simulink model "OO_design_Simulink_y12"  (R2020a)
settings: Solver=ode45  StartTime=0.0  StopTime=100  RelTol=1e-3  EnableMultiTasking=on
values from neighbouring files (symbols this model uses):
  Ao1 = Am-K1*Cm(1,:)    [OO_design.m]    (also in OO_design_y12.m = Am - K1*Cm(1,:))
  Ao2 = Am-K2*Cm(2,:)    [OO_design.m]    (also in OO_design_y12.m = Am - K2*Cm(2,:))
  Bo1 = [Bm K1]    [OO_design.m]    (also in OO_design_y12.m)
  Bo2 = [Bm-K2*Dm(2,1) K2]    [OO_design.m]    (also in OO_design_y12.m)
  Co1 = Cm(1,:)    [OO_design.m]    (also in OO_design_y12.m)
  Co2 = Cm(2,:)    [OO_design.m]    (also in OO_design_y12.m)
  Do1 = zeros(1,2)    [OO_design.m]    (also in OO_design_y12.m)
  Do2 = [Dm(2,1) 0]    [OO_design.m]    (also in OO_design_y12.m)
  Ts = 0.05    [init_model.m]

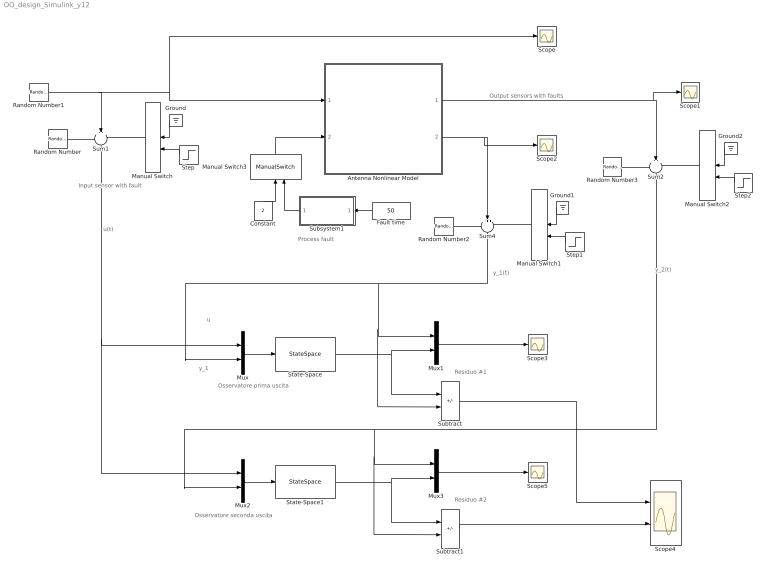
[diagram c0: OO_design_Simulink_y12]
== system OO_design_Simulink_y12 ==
  note: Osservatore seconda uscita
  note: Residuo #2
  note: Residuo #1
  note: Osservatore prima uscita
  note: y_1
  note: u
  note: u(t)
  note: Output sensors with faults
  note: Process fault
  note: Input sensor with fault
  note: y_1(t)
  note: y_2(t)
  Antenna Nonlinear Model : Subsystem
  Constant : Constant  Value=2
  Fault time : Constant  Value=50
  Ground : Ground
  Ground1 : Ground
  Ground2 : Ground
  Manual Switch{,1..3} (4 alike) : ManualSwitch
  Mux{,1..3} (4 alike) : Mux  Inputs=2
  Random Number : RandomNumber  Variance=0.0001  Seed=1  SampleTime=Ts
  Random Number1 : RandomNumber  Variance=0.1  SampleTime=10
  Random Number2 : RandomNumber  Variance=0.00001  Seed=2  SampleTime=Ts
  Random Number3 : RandomNumber  Variance=0.00001  Seed=3  SampleTime=Ts
  Scope{,1..3,5} (5 alike) : Scope
  Scope4 : Scope  NumInputPorts=2
  State-Space : StateSpace  A=Ao1  B=Bo1  C=Co1  D=Do1  InitialCondition=0
  State-Space1 : StateSpace  A=Ao2  B=Bo2  C=Co2  D=Do2  InitialCondition=0
  Step : Step  Time=50  SampleTime=0
  Step1 : Step  Time=50  SampleTime=0
  Step2 : Step  Time=50  SampleTime=0
  Subsystem1 : Subsystem
  Subtract : Sum  Inputs=+-
  Subtract1 : Sum  Inputs=+-
  Sum1 : Sum  Inputs=+++  SaturateOnIntegerOverflow=on
  Sum2 : Sum  Inputs=+++  SaturateOnIntegerOverflow=on
  Sum4 : Sum  Inputs=+++  SaturateOnIntegerOverflow=on
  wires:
  Random Number1/1 -> Scope/1, Antenna Nonlinear Model/1(force), Sum1/2
  Random Number/1 -> Sum1/1
  Manual Switch/1 -> Sum1/3
  Sum1/1 -> Mux2/1, Mux/1
  Ground/1 -> Manual Switch/1
  Step/1 -> Manual Switch/2
  Random Number2/1 -> Sum4/1
  Sum4/1 -> Mux1/1, Subtract/2, Mux/2
  Ground1/1 -> Manual Switch1/1
  Manual Switch1/1 -> Sum4/3
  Step1/1 -> Manual Switch1/2
  Antenna Nonlinear Model/2(velocity) -> Sum4/2, Scope2/1
  Random Number3/1 -> Sum2/1
  Ground2/1 -> Manual Switch2/1
  Manual Switch2/1 -> Sum2/3
  Step2/1 -> Manual Switch2/2
  Antenna Nonlinear Model/1(angle) -> Sum2/2, Scope1/1
  Sum2/1 -> Mux3/1, Subtract1/2, Mux2/2
  Fault time/1 -> Subsystem1/1(Fault time)
  Subsystem1/1(Fault) -> Manual Switch3/2
  Manual Switch3/1 -> Antenna Nonlinear Model/2(drag)
  Constant/1 -> Manual Switch3/1
  Mux/1 -> State-Space/1
  State-Space/1 -> Subtract/1, Mux1/2
  Subtract/1 -> Scope4/1
  Mux1/1 -> Scope3/1
  Mux2/1 -> State-Space1/1
  State-Space1/1 -> Subtract1/1, Mux3/2
  Mux3/1 -> Scope5/1
  Subtract1/1 -> Scope4/2

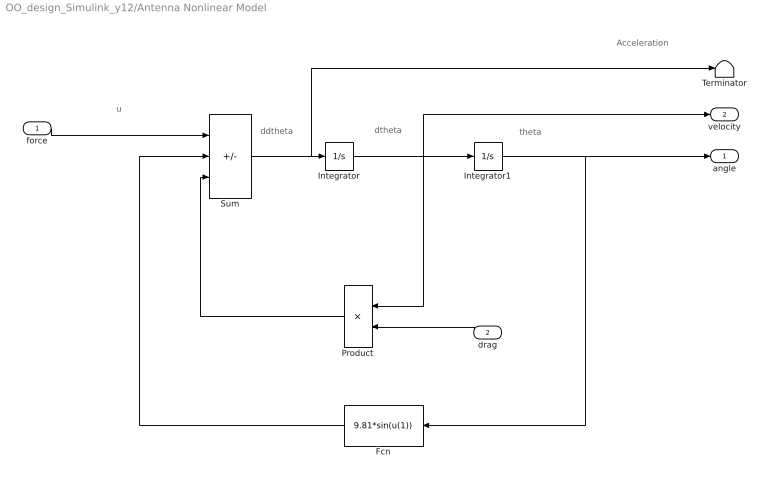
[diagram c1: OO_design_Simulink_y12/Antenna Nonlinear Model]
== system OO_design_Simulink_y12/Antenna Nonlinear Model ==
  note: Acceleration
  note: ddtheta
  note: dtheta
  note: theta
  note: u
  force : Inport
  drag : Inport  Port=2
  Fcn : Fcn  Expr=9.81*sin(u(1))
  Integrator : Integrator
  Integrator1 : Integrator  InitialCondition=(pi/180)*90
  Product : Product
  Sum : Sum  Inputs=+--  SaturateOnIntegerOverflow=on
  Terminator : Terminator
  angle : Outport
  velocity : Outport  Port=2
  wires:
  Sum/1 -> Terminator/1, Integrator/1
  Integrator/1 -> Product/1, Integrator1/1, velocity/1
  Integrator1/1 -> angle/1, Fcn/1
  Fcn/1 -> Sum/2
  Product/1 -> Sum/3
  force/1 -> Sum/1
  drag/1 -> Product/2

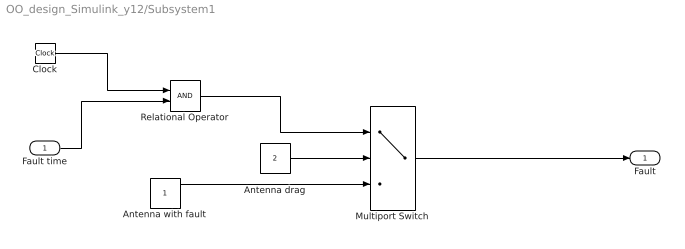
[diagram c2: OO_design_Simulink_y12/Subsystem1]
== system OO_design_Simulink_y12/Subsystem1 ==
  Fault time : Inport
  Antenna drag : Constant  Value=2
  Antenna with fault : Constant
  Clock : Clock
  Multiport Switch : MultiPortSwitch  DataPortOrder=Zero-based contiguous  Inputs=2  zeroidx=on
  Relational Operator : RelationalOperator  OutDataTypeStr=boolean  RndMeth=Simplest
  Fault : Outport
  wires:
  Clock/1 -> Relational Operator/1
  Fault time/1 -> Relational Operator/2
  Antenna drag/1 -> Multiport Switch/2
  Relational Operator/1 -> Multiport Switch/1
  Multiport Switch/1 -> Fault/1
  Antenna with fault/1 -> Multiport Switch/3
